| IBIS file stm32l552_562_ufbga132.ibs
[IBIS ver]   4.2
[File name]  stm32l552_562_ufbga132.ibs
[File Rev]   1.0
[Date]   04-10-2019
[Source]   Data Created at STMicroelectronics
[Notes]   File originated from ELDO simulations.
[Disclaimer] This information is for modeling purpose only and is
   not guaranted.
   The information is subject to change without notice.
[Copyright]  Copyright 2019 STMicroelectronics Inc.
|   Component stm32l552_562_ufbga132
[Component] stm32l552_562_ufbga132
[Manufacturer] STMicroelectronics
[Package]
| variable   typ   min   max
R_pkg  0  NA  NA
L_pkg  0  NA  NA
C_pkg  0  NA  NA
[Pin]   signal_name   model_name R_pin L_pin C_pin
A1 PE5 io8prog2m25m50m120m_sudq_ft
A10 PC11 io8prog2m25m50m120m_sudq_ft
A11 PA15 io6usb_bmc_pd_cc_ft
A12 VDDUSB POWER
A2 PE3 io8prog2m25m50m120m_sudq_ft
A3 PE1 io8prog2m25m50m120m_sudq_ft
A4 PB9 io8prog2m25m50m120m_sudq_i2c_ft
A5 PB6 io8prog2m25m50m120m_sudq_i2c_ft
A6 PG12 io8prog2m25m50m120m_sudq_ft
A7 PD6 io8prog2m25m50m120m_sudq_ft
A8 PD5 io8prog2m25m50m120m_sudq_ft
A9 PD2 io8prog2m25m50m120m_sudq_ft
B1 VBAT POWER
B10 PC12 io8prog2m25m50m120m_sudq_ft
B11 PC10 io8prog2m25m50m120m_sudq_ft
B12 PA12 io8usblsfs_otg2
B2 PE4 io8prog2m25m50m120m_sudq_ft
B3 PE2 io8prog2m25m50m120m_sudq_ft
B4 PG15 io8prog2m25m50m120m_sudq_ft
B5 PH3-BOOT0 io8prog2m25m50m120m_sudq_ft
B6 PB4 io8prog2m25m50m120m_sudq_i2c_ft
B7 PG9 io8prog2m25m50m120m_sudq_ft
B8 PD4 io8prog2m25m50m120m_sudq_ft
B9 PD1 io8prog2m25m50m120m_sudq_ft
C1 PC14-OSC32_IN io8prog2m25m50m120m_sudq_ft
C10 PA13 io8prog2m25m50m120m_sudq_ft
C11 PA14 io8prog2m25m50m120m_sudq_i2c_ft
C12 PA11 io8usblsfs_otg2
C2 PE6 io8prog2m25m50m120m_sudq_ft
C3 PC13 io8prog2m25m50m120m_sudq_ft
C4 PE0 io8prog2m25m50m120m_sudq_ft
C5 PB8 io8prog2m25m50m120m_sudq_i2c_ft
C6 PB3 io8prog2m25m50m120m_sudq_ft
C7 PG10 io8prog2m25m50m120m_sudq_ft
C8 PD3 io8prog2m25m50m120m_sudq_ft
C9 PD0 io8prog2m25m50m120m_sudq_ft
D1 PC15-OSC32_OUT io8prog2m25m50m120m_sudq_ft
D10 PA9 io8prog2m25m50m120m_sudq_ft
D11 PA10 io8prog2m25m50m120m_sudq_ft
D12 PA8 io8prog2m25m50m120m_sudq_i2c_ft
D2 PF0 io8prog2m25m50m120m_sudq_i2c_ft
D3 PF3 io8prog2m25m50m120m_sudq_ft
D4 VDD POWER
D5 PB7 io8prog2m25m50m120m_sudq_i2c_ft
D6 PB5 io8prog2m25m50m120m_sudq_ft
D7 PD7 io8prog2m25m50m120m_sudq_ft
D8 VDDIO2 POWER
D9 VDD POWER
E1 PF2 io8prog2m25m50m120m_sudq_ft
E10 PC7 io8prog2m25m50m120m_sudq_ft
E11 PC9 io8prog2m25m50m120m_sudq_i2c_ft
E12 PC8 io8prog2m25m50m120m_sudq_ft
E2 PF1 io8prog2m25m50m120m_sudq_i2c_ft
E3 PF4 io8prog2m25m50m120m_sudq_ft
E4 VSS GND
E9 VSS GND
F1 PH0-OSC_IN io8prog2m25m50m120m_sudq_ft
F10 PG7 io8prog2m25m50m120m_sudq_i2c_ft
F11 PC6 io8prog2m25m50m120m_sudq_ft
F12 PG8 io8prog2m25m50m120m_sudq_i2c_ft
F2 PF5 io8prog2m25m50m120m_sudq_ft
F3 PC2 io8prog2m25m50m120m_sudq_ft
F4 PC3 io8prog2m25m50m120m_sudq_ft
F6 VSS GND
F7 VDD POWER
F9 PG6 io8prog2m25m50m120m_sudq_ft
G1 PH1-OSC_OUT io8prog2m25m50m120m_sudq_ft
G10 PG2 io8prog2m25m50m120m_sudq_ft
G11 PG3 io8prog2m25m50m120m_sudq_ft
G12 PG5 io8prog2m25m50m120m_sudq_ft
G2 NRST ioreset_ft_v33
G3 PC1 io8prog2m25m50m120m_sudq_i2c_ft
G4 PA1 io8prog2m25m50m120m_sudq_ft
G6 VDD POWER
G7 VSS GND
G9 PG4 io8prog2m25m50m120m_sudq_ft
H1 VSSA_VREF- GND
H3  OPAMP1_VINM NC
H10 PD14 io8prog2m25m50m120m_sudq_ft
H11 PD13 io8prog2m25m50m120m_sudq_i2c_ft
H12 PD15 io8prog2m25m50m120m_sudq_ft
H2 PC0 io8prog2m25m50m120m_sudq_i2c_ft
H4 VSS GND
H9 VSS GND
J1 VREF+ POWER
J10 PD9 io8prog2m25m50m120m_sudq_ft
J11 PD11 io8prog2m25m50m120m_sudq_ft
J12 PD12 io8prog2m25m50m120m_sudq_i2c_ft
J2 PA0 io8prog2m25m50m120m_sudq_ft
J3 PC5 io8prog2m25m50m120m_sudq_ft
J4 VDD POWER
J5 PF14 io8prog2m25m50m120m_sudq_i2c_ft
J6 PE8 io8prog2m25m50m120m_sudq_ft
J7 PE10 io8prog2m25m50m120m_sudq_ft
J8 PE12 io8prog2m25m50m120m_sudq_ft
J9 VDD POWER
K1 VDDA POWER
K10 PB13 io8prog2m25m50m120m_sudq_i2c_ft
K11 PB14 io8prog2m25m50m120m_sudq_i2c_ft
K12 PB15 io6usb_bmc_pd_cc_ft
K2 PA2 io8prog2m25m50m120m_sudq_ft
K3 PA7 io8prog2m25m50m120m_sudq_i2c_ft
K4 PB2 io8prog2m25m50m120m_sudq_ft
K5 PF11 io8prog2m25m50m120m_sudq_ft
K6 PG1 io8prog2m25m50m120m_sudq_ft
K7 PE7 io8prog2m25m50m120m_sudq_ft
K8 PE14 io8prog2m25m50m120m_sudq_ft
K9 PB10 io8prog2m25m50m120m_sudq_i2c_ft
L1 PA3 io8prog2m25m50m120m_sudq_ft
L10 VSS GND
L11 PB12 io8prog2m25m50m120m_sudq_ft
L12 PD8 io8prog2m25m50m120m_sudq_ft
L2 PA6 io8prog2m25m50m120m_sudq_ft
L3 PA4 io8prog2m25m50m120m_sudq_ft
L4 PB1 io8prog2m25m50m120m_sudq_ft
L5 PF12 io8prog2m25m50m120m_sudq_ft
L6 PF15 io8prog2m25m50m120m_sudq_i2c_ft
L7 PE11 io8prog2m25m50m120m_sudq_ft
L8 PE15 io8prog2m25m50m120m_sudq_ft
L9 PB11 io8prog2m25m50m120m_sudq_i2c_ft
M1 PA5 io8prog2m25m50m120m_sudq_ft
M10 PG13 io8prog2m25m50m120m_sudq_i2c_ft
M11 PG11 io8prog2m25m50m120m_sudq_ft
M12 PD10 io8prog2m25m50m120m_sudq_ft
M2 OPAMP2_VINM NC
M3 PC4 io8prog2m25m50m120m_sudq_ft
M4 PB0 io8prog2m25m50m120m_sudq_ft
M5 PF13 io8prog2m25m50m120m_sudq_ft
M6 PG0 io8prog2m25m50m120m_sudq_ft
M7 PE9 io8prog2m25m50m120m_sudq_ft
M8 PE13 io8prog2m25m50m120m_sudq_ft
M9 PG14 io8prog2m25m50m120m_sudq_i2c_ft
[Model Selector] io6usb_bmc_pd_cc_ft
usb_bmc_emit_pdccpd  "BMC PD emitter  + PD"
usb_bmc_emit_pdcc3a0  "BMC PD emitter  + 3rd PU"
usb_bmc_emit_pdcc1a5  "BMC PD emitter  + 2nd PU"
usb_bmc_emit_pdccusb  "BMC PD emitter  + 1st PU"
usb_bmc_emit  "BMC PD emitter "
io2_pdcc_ft_3v3_lowspeed  "GPIO-3.3V range - low speed"
io2_pdcc_ft_3v3_mediumspeed  "GPIO-3.3V range - medium speed"
io2_pdcc_ft_3v3_lowspeed_pu  "GPIO-3.3V range - low speed - pull up"
io2_pdcc_ft_3v3_mediumspeed_pu  "GPIO-3.3V range - medium speed - pull up"
io2_pdcc_ft_3v3_lowspeed_pd  "GPIO-3.3V range - low speed - pull down"
io2_pdcc_ft_3v3_mediumspeed_pd  "GPIO-3.3V range - medium speed - pull down"
io2_pdcc_ft_1v8_lowspeed  "GPIO-1.8V range - low speed"
io2_pdcc_ft_1v8_mediumspeed  "GPIO-1.8V range - medium speed"
io2_pdcc_ft_1v8_lowspeed_pu  "GPIO-1.8V range - low speed - pull up"
io2_pdcc_ft_1v8_mediumspeed_pu  "GPIO-1.8V range - medium speed - pull up"
io2_pdcc_ft_1v8_lowspeed_pd  "GPIO-1.8V range - low speed - pull down"
io2_pdcc_ft_1v8_mediumspeed_pd  "GPIO-1.8V range - medium speed - pull down"
io2_pdcc_ft_1v2_lowspeed  "GPIO-1.2V range - low speed"
io2_pdcc_ft_1v2_mediumspeed  "GPIO-1.2V range - medium speed"
io2_pdcc_ft_1v2_lowspeed_pu  "GPIO-1.2V range - low speed - pull up"
io2_pdcc_ft_1v2_mediumspeed_pu  "GPIO-1.2V range - medium speed - pull up"
io2_pdcc_ft_1v2_lowspeed_pd  "GPIO-1.2V range - low speed - pull down"
io2_pdcc_ft_1v2_mediumspeed_pd  "GPIO-1.2V range - medium speed - pull down"
[Model Selector] io8prog2m25m50m120m_sudq_ft
iols8p_sudq_ft_pd_lv  "IO low speed, PD=40kOhm - 1P8V"
iols8p_sudq_ft_pu_lv  "IO low speed, PU=40kOhm - 1P8V"
iols8p_sudq_ft_lv  "IO low speed - 1P8V"
iols8p_sudq_ft_pd  "IO low speed, PD=40kOhm - 3P3V"
iols8p_sudq_ft_pu  "IO low speed, PU=40kOhm - 3P3V"
iols8p_sudq_ft  "IO low speed - 3P3V"
iofs8p_sudq_ft_pd_lv  "IO full speed, PD=40kOhm - 1P8V"
iofs8p_sudq_ft_pu_lv  "IO full speed, PU=40kOhm - 1P8V"
iofs8p_sudq_ft_lv  "IO full speed - 1P8V"
iofs8p_sudq_ft_pd  "IO full speed, PD=40kOhm - 3P3V"
iofs8p_sudq_ft_pu  "IO full speed, PU=40kOhm - 3P3V"
iofs8p_sudq_ft  "IO full speed - 3P3V"
ioms8p_sudq_ft_pd_lv  "IO medium speed, PD=40kOhm - 1P8V"
ioms8p_sudq_ft_pu_lv  "IO medium speed, PU=40kOhm - 1P8V"
ioms8p_sudq_ft_lv  "IO medium speed - 1P8V"
ioms8p_sudq_ft_pd  "IO medium speed, PD=40kOhm - 3P3V"
ioms8p_sudq_ft_pu  "IO medium speed, PU=40kOhm - 3P3V"
ioms8p_sudq_ft  "IO medium speed - 3P3V"
iohs8p_sudq_ft_pd_lv  "IO high speed, PD=40kOhm - 1P8V"
iohs8p_sudq_ft_pu_lv  "IO high speed, PU=40kOhm - 1P8V"
iohs8p_sudq_ft_lv  "IO high speed - 1P8V"
iohs8p_sudq_ft_pd  "IO high speed, PD=40kOhm - 3P3V"
iohs8p_sudq_ft_pu  "IO high speed, PU=40kOhm - 3P3V"
iohs8p_sudq_ft  "IO high speed - 3P3V"
[Model Selector] io8prog2m25m50m120m_sudq_i2c_ft
io8prog_1v8_i2c_pd  "5V Tol GPIO 1.8V range i2c functionality with pull down"
io8prog_1v8_i2c_pu  "5V Tol GPIO 1.8V range i2c functionality with pull up"
io8prog_1v8_i2c  "5V Tol GPIO 1.8V range i2c functionality"
io8prog_3v3_i2c_pd  "5V Tol GPIO 3.3V range i2c functionality with pull down"
io8prog_3v3_i2c_pu  "5V Tol GPIO 3.3V range i2c functionality with pull up"
io8prog_3v3_i2c  "5V Tol GPIO 3.3V range i2c functionality"
iols8p_sudq_ft_pd_lv  "IO low speed, PD=40kOhm - 1P8V"
iols8p_sudq_ft_pu_lv  "IO low speed, PU=40kOhm - 1P8V"
iols8p_sudq_ft_lv  "IO low speed - 1P8V"
iols8p_sudq_ft_pd  "IO low speed, PD=40kOhm - 3P3V"
iols8p_sudq_ft_pu  "IO low speed, PU=40kOhm - 3P3V"
iols8p_sudq_ft  "IO low speed - 3P3V"
iofs8p_sudq_ft_pd_lv  "IO full speed, PD=40kOhm - 1P8V"
iofs8p_sudq_ft_pu_lv  "IO full speed, PU=40kOhm - 1P8V"
iofs8p_sudq_ft_lv  "IO full speed - 1P8V"
iofs8p_sudq_ft_pd  "IO full speed, PD=40kOhm - 3P3V"
iofs8p_sudq_ft_pu  "IO full speed, PU=40kOhm - 3P3V"
iofs8p_sudq_ft  "IO full speed - 3P3V"
ioms8p_sudq_ft_pd_lv  "IO medium speed, PD=40kOhm - 1P8V"
ioms8p_sudq_ft_pu_lv  "IO medium speed, PU=40kOhm - 1P8V"
ioms8p_sudq_ft_lv  "IO medium speed - 1P8V"
ioms8p_sudq_ft_pd  "IO medium speed, PD=40kOhm - 3P3V"
ioms8p_sudq_ft_pu  "IO medium speed, PU=40kOhm - 3P3V"
ioms8p_sudq_ft  "IO medium speed - 3P3V"
iohs8p_sudq_ft_pd_lv  "IO high speed, PD=40kOhm - 1P8V"
iohs8p_sudq_ft_pu_lv  "IO high speed, PU=40kOhm - 1P8V"
iohs8p_sudq_ft_lv  "IO high speed - 1P8V"
iohs8p_sudq_ft_pd  "IO high speed, PD=40kOhm - 3P3V"
iohs8p_sudq_ft_pu  "IO high speed, PU=40kOhm - 3P3V"
iohs8p_sudq_ft  "IO high speed - 3P3V"
[Model Selector] io8usblsfs_otg2
usb_ls_pd  "USB Low Speed mode - Pull Down"
usb_ls_pu2  "USB Low Speed mode - Pull up 2"
usb_ls_pu  "USB Low Speed mode - Pull up"
usb_fs  "USB Low Speed mode"
usb_fs_pd  "USB Full Speed mode - Pull Down"
usb_fs_pu2  "USB Full Speed mode - Pull up 2"
usb_fs_pu  "USB Full Speed mode - Pull up"
[Model Selector] ioreset_ft_v33
ioreset_1v2_pu  "RESET 1.2V range with PU"
ioreset_1v2  "RESET 1.2V range"
ioreset_1v8_pu  "RESET 1.8V range with PU"
ioreset_1v8  "RESET 1.8V range"
ioreset_3v3_pu  "RESET 3.3V range with PU"
ioreset_3v3  "RESET 3.3V range"
| Models and submodels in the file (66): usb_bmc_emit_pdccpd (I/O), usb_bmc_emit_pdcc3a0 (I/O), usb_bmc_emit_pdcc1a5 (I/O), usb_bmc_emit_pdccusb (I/O), usb_bmc_emit (I/O), io2_pdcc_ft_3v3_lowspeed (I/O), io2_pdcc_ft_3v3_mediumspeed (I/O), io2_pdcc_ft_3v3_lowspeed_pu (I/O), io2_pdcc_ft_3v3_mediumspeed_pu (I/O), io2_pdcc_ft_3v3_lowspeed_pd (I/O), io2_pdcc_ft_3v3_mediumspeed_pd (I/O), io2_pdcc_ft_1v8_lowspeed (I/O), io2_pdcc_ft_1v8_mediumspeed (I/O), io2_pdcc_ft_1v8_lowspeed_pu (I/O), io2_pdcc_ft_1v8_mediumspeed_pu (I/O), io2_pdcc_ft_1v8_lowspeed_pd (I/O), io2_pdcc_ft_1v8_mediumspeed_pd (I/O), io2_pdcc_ft_1v2_lowspeed (I/O), io2_pdcc_ft_1v2_mediumspeed (I/O), io2_pdcc_ft_1v2_lowspeed_pu (I/O), io2_pdcc_ft_1v2_mediumspeed_pu (I/O), io2_pdcc_ft_1v2_lowspeed_pd (I/O), io2_pdcc_ft_1v2_mediumspeed_pd (I/O), iols8p_sudq_ft_pd_lv (I/O), iols8p_sudq_ft_pu_lv (I/O), iols8p_sudq_ft_lv (I/O), iols8p_sudq_ft_pd (I/O), iols8p_sudq_ft_pu (I/O), iols8p_sudq_ft (I/O), iofs8p_sudq_ft_pd_lv (I/O), iofs8p_sudq_ft_pu_lv (I/O), iofs8p_sudq_ft_lv (I/O), iofs8p_sudq_ft_pd (I/O), iofs8p_sudq_ft_pu (I/O), iofs8p_sudq_ft (I/O), ioms8p_sudq_ft_pd_lv (I/O), ioms8p_sudq_ft_pu_lv (I/O), ioms8p_sudq_ft_lv (I/O), ioms8p_sudq_ft_pd (I/O), ioms8p_sudq_ft_pu (I/O), ioms8p_sudq_ft (I/O), iohs8p_sudq_ft_pd_lv (I/O), iohs8p_sudq_ft_pu_lv (I/O), iohs8p_sudq_ft_lv (I/O), iohs8p_sudq_ft_pd (I/O), iohs8p_sudq_ft_pu (I/O), iohs8p_sudq_ft (I/O), io8prog_1v8_i2c_pd (I/O_open_drain), io8prog_1v8_i2c_pu (I/O_open_drain), io8prog_1v8_i2c (I/O_open_drain), io8prog_3v3_i2c_pd (I/O_open_drain), io8prog_3v3_i2c_pu (I/O_open_drain), io8prog_3v3_i2c (I/O_open_drain), usb_ls_pd (I/O), usb_ls_pu2 (I/O), usb_ls_pu (I/O), usb_fs (I/O), usb_fs_pd (I/O), usb_fs_pu2 (I/O), usb_fs_pu (I/O), ioreset_1v2_pu (I/O_open_drain), ioreset_1v2 (I/O_open_drain), ioreset_1v8_pu (I/O_open_drain), ioreset_1v8 (I/O_open_drain), ioreset_3v3_pu (I/O_open_drain), ioreset_3v3 (I/O_open_drain)
